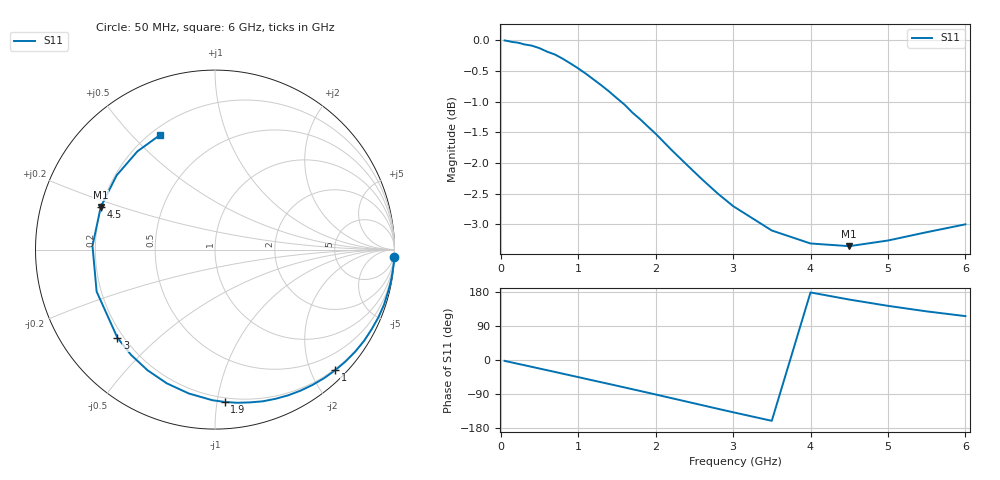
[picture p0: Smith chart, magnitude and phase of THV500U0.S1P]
! SIEMENS Discrete & RF Semiconductors
! BAS70
! Si Schottky Diode in SOT23
! VR = 0.5 V
! S-Parameters:  February  1997
# GHz  S  MA  R  50
!  f  S11
! GHz  MAG  ANG
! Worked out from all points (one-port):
!   34 points, 50 MHz to 6 GHz, reference 50 ohm
!   lowest |S11| = -3.4 dB at 4.5 GHz (marker M1), VSWR 5.24, Z = 9.84 + j8.7 ohm
!   |S11| at or under -10 dB: nowhere
!   S11 on the Smith chart (normalised r, x): 50 MHz: 0, -50; 1 GHz: 0.18, -2.40; 1.9 GHz: 0.17, -1.05; 3 GHz: 0.18, -0.37; 4.5 GHz: 0.20, +0.17; 6 GHz: 0.24, +0.60
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0.05  1 -2.3
0.25  0.9949 -11.3
0.4  0.9903 -18.0
0.5  0.9856 -22.5
0.6  0.9791 -27.0
0.7  0.9739 -31.5
0.8  0.9663 -36.1
1  0.9489 -45.1
1.1  0.9394 -49.7
1.2  0.9292 -54.3
1.3  0.9191 -58.8
1.4  0.9085 -63.3
1.5  0.8971 -67.9
1.6  0.8862 -72.5
1.8  0.8625 -81.7
1.9  0.8507 -86.3
2  0.8393 -91.0
2.2  0.8147 -100.4
2.4  0.792 -109.8
2.6  0.7703 -119.2
2.8  0.7503 -128.6
3  0.7326 -137.9
3.5  0.6997 -160.5
4  0.6829 178.3
4.5  0.6794 159.5
5  0.6867 142.9
5.5  0.6975 128.3
6  0.7079 115.8
